(* Logix 5000 Controller export Example_PLC; controller Example_PLC 1769-L32E rev 19.11; software revision 19.01; part 6 of 6 *)

ADD_ON_INSTRUCTION AKD_Stop_Smooth   (* revision 2.3, ExecutePrescan, ExecuteEnableInFalse *)
// Motion Smooth Stop
// Revision note:
// Remove the command timeout (allow unlimited time to stop). Add an IP In Progress bit which is active while stopping.
VAR_OUTPUT
   DN : BOOL; {access Read Only, visible}   // Command Successful
   ER : BOOL; {access Read Only, visible}   // Error
END_VAR
VAR_IN_OUT
   Axis : AKD_Axis; {required}
END_VAR
VAR_OUTPUT
   IP : BOOL; {access Read Only, visible}   // In Progress
END_VAR

ROUTINE EnableInFalse   (* ladder *)
// Enable In False
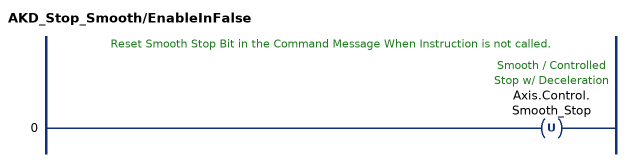
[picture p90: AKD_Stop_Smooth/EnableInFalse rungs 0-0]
   // Reset Smooth Stop Bit in the Command Message When Instruction is not called.
   0: OTU(Axis.Control.Smooth_Stop);
END_ROUTINE

ROUTINE Logic   (* ladder *)
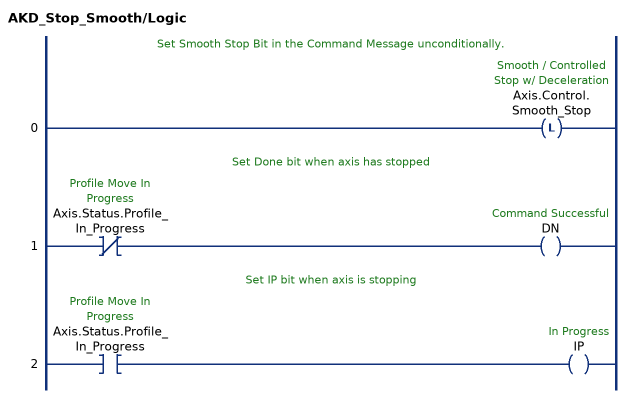
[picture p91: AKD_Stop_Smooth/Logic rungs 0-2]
   // Set Smooth Stop Bit in the Command Message unconditionally.
   0: OTL(Axis.Control.Smooth_Stop);
   // Set Done bit when axis has stopped
   1: XIO(Axis.Status.Profile_In_Progress)OTE(DN);
   // Set IP bit when axis is stopping
   2: XIC(Axis.Status.Profile_In_Progress)OTE(IP);
END_ROUTINE

ROUTINE Prescan   (* ladder *)
END_ROUTINE
END_ADD_ON_INSTRUCTION

ADD_ON_INSTRUCTION AKD_Torque_Move   (* revision 2.1, ExecutePrescan, ExecuteEnableInFalse *)
// Set Torque Command
VAR_OUTPUT
   DN : BOOL; {access Read Only, visible}   // Command Successful
   ER : BOOL; {access Read Only, visible}   // Error
END_VAR
VAR_IN_OUT
   Axis : AKD_Axis; {required}
END_VAR
VAR_INPUT
   Torque : DINT; {required}   // Torque Command
END_VAR
VAR
   Response_Bytes : SINT[8];
   OS_LoadStart : BOOL;
   Command_Timeout : TIMER := (PRE := 100);   // Timeout Timer
   Command_Message_Type : SINT;   // Command Message Type
   Command_Axis_Number : SINT;   // Command Axis Number
   Response_Message_Type : SINT;   // Response Message Type
   Response_Axis_Number : SINT;   // Response Axis Number
   Command_Bytes : SINT[8];
   Step : SINT;
END_VAR

ROUTINE EnableInFalse   (* ladder *)
// EnableIn_False
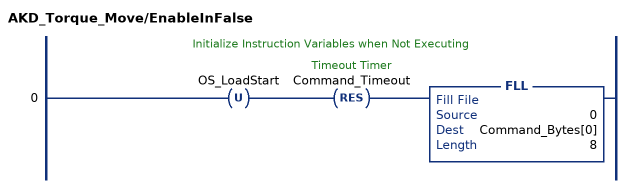
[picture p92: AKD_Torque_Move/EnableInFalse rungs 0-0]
   // Initialize Instruction Variables when Not Executing
   0: OTU(OS_LoadStart)RES(Command_Timeout)FLL(0,Command_Bytes[0],8);
END_ROUTINE

ROUTINE Logic   (* ladder *)
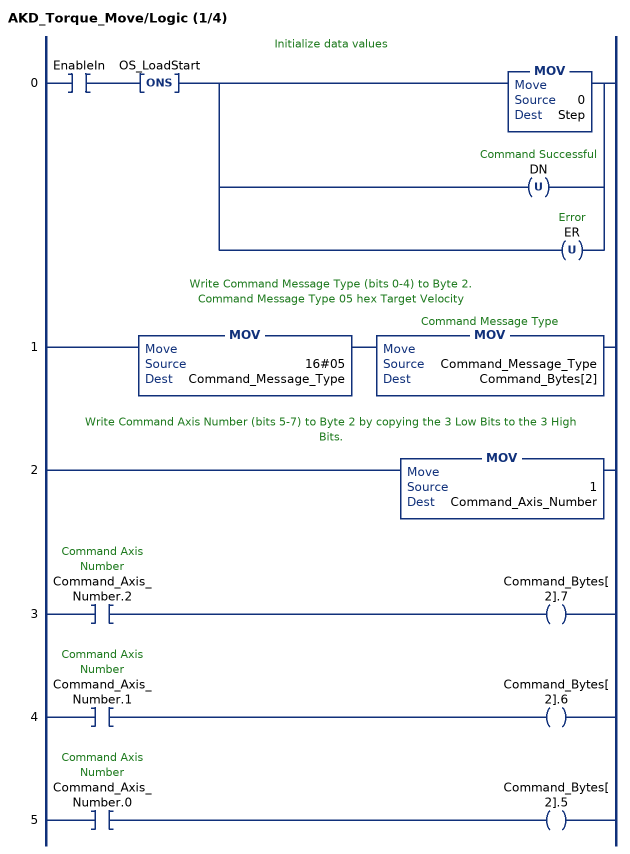
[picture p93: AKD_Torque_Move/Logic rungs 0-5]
   // Initialize data values
   0: XIC(EnableIn)ONS(OS_LoadStart)[MOV(0,Step) ,OTU(DN) ,OTU(ER) ];
   // Write Command Message Type (bits 0-4) to Byte 2.
   // Command Message Type 05 hex Target Velocity
   1: MOV(16#05,Command_Message_Type)MOV(Command_Message_Type,Command_Bytes[2]);
   // Write Command Axis Number (bits 5-7) to Byte 2 by copying the 3 Low Bits to the 3 High Bits.
   2: MOV(1,Command_Axis_Number);
   3: XIC(Command_Axis_Number.2)OTE(Command_Bytes[2].7);
   4: XIC(Command_Axis_Number.1)OTE(Command_Bytes[2].6);
   5: XIC(Command_Axis_Number.0)OTE(Command_Bytes[2].5);
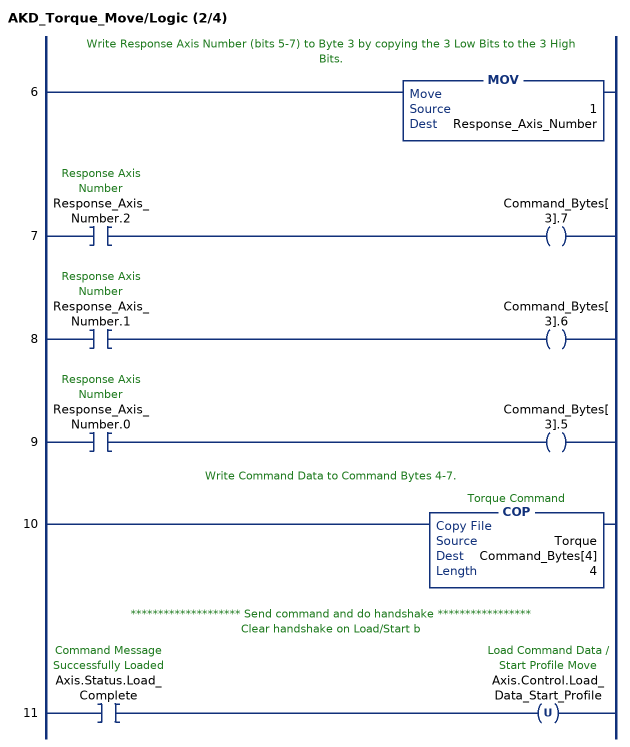
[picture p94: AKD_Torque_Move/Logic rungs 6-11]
   // Write Response Axis Number (bits 5-7) to Byte 3 by copying the 3 Low Bits to the 3 High Bits.
   6: MOV(1,Response_Axis_Number);
   7: XIC(Response_Axis_Number.2)OTE(Command_Bytes[3].7);
   8: XIC(Response_Axis_Number.1)OTE(Command_Bytes[3].6);
   9: XIC(Response_Axis_Number.0)OTE(Command_Bytes[3].5);
   // Write Command Data to Command Bytes 4-7.
   10: COP(Torque,Command_Bytes[4],4);
   // ******************** Send command and do handshake *****************
   // Clear handshake on Load/Start b
   11: XIC(Axis.Status.Load_Complete)OTU(Axis.Control.Load_Data_Start_Profile);
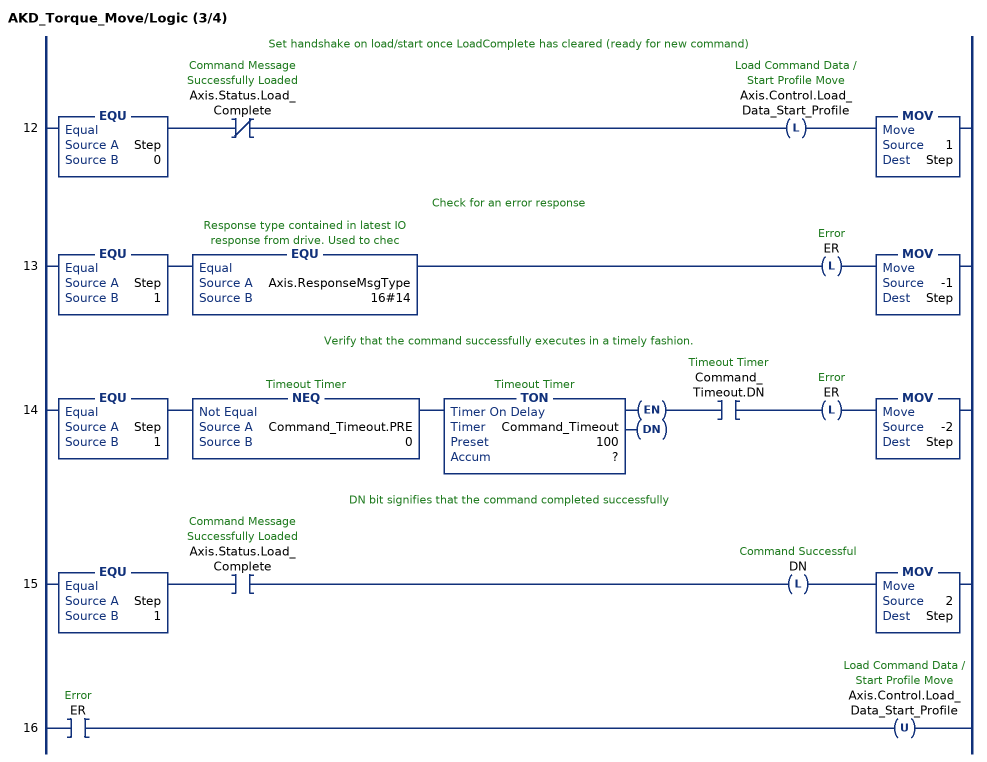
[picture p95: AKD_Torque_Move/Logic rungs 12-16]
   // Set handshake on load/start once LoadComplete has cleared (ready for new command)
   12: EQU(Step,0)XIO(Axis.Status.Load_Complete)OTL(Axis.Control.Load_Data_Start_Profile)MOV(1,Step);
   // Check for an error response
   13: EQU(Step,1)EQU(Axis.ResponseMsgType,16#14)OTL(ER)MOV(-1,Step);
   // Verify that the command successfully executes in a timely fashion.
   14: EQU(Step,1)NEQ(Command_Timeout.PRE,0)TON(Command_Timeout,?,?)XIC(Command_Timeout.DN)OTL(ER)MOV(-2,Step);
   // DN bit signifies that the command completed successfully
   15: EQU(Step,1)XIC(Axis.Status.Load_Complete)OTL(DN)MOV(2,Step);
   16: XIC(ER)OTU(Axis.Control.Load_Data_Start_Profile);
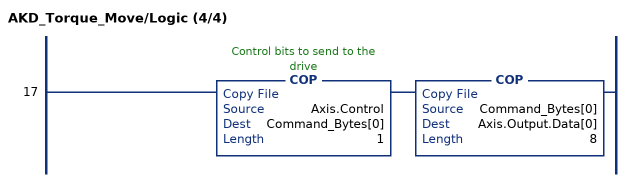
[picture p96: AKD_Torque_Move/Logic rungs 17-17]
   17: COP(Axis.Control,Command_Bytes[0],1)COP(Command_Bytes[0],Axis.Output.Data[0],8);
END_ROUTINE

ROUTINE Prescan   (* ladder *)
// Prescan
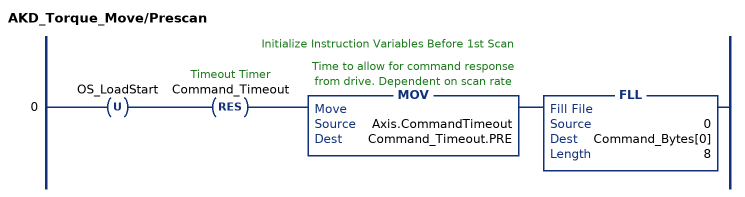
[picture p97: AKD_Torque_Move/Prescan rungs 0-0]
   // Initialize Instruction Variables Before 1st Scan
   0: OTU(OS_LoadStart)RES(Command_Timeout)MOV(Axis.CommandTimeout,Command_Timeout.PRE)FLL(0,Command_Bytes[0],8);
END_ROUTINE
END_ADD_ON_INSTRUCTION

VAR_GLOBAL   (* controller tags *)
   AIN_VALUE : DINT := 7047;
   AKD_1 : AKD_Drive;
   AOUT : DINT;
   AOUT_VALUEU : LINT;
   Axis_1 : AKD_Drive;
   AXIS_ONE : AKD_Axis := (Status.Current_Direction := 1, Input.Data[0] := 16, Input.Data[8] := -6, Input.Data[9] := 78, Input.Data[12] := -19, Input.Data[13] := 10, PositionFeedback := 20218, VelocityFeedback := 2797);
   DIN1_STATE : BOOL;
   DM_EN_SET : BOOL := 1;
   DOUT_STATEU : BOOL;
   Dynamic : BOOL;
   EN : BOOL;
   OneShot : BOOL;
   Start_Dynamic_data_transfer : BOOL;
   Start_Dynamic_mapped_Data : BOOL;
END_VAR

PROGRAM MainProgram   (* main routine MainRoutine *)

ROUTINE MainRoutine   (* ladder *)
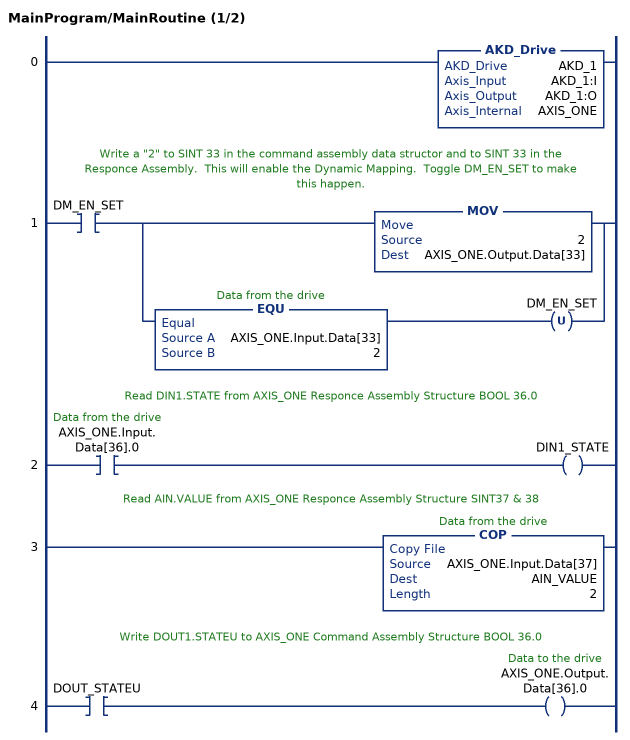
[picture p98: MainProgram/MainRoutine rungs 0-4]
   0: AKD_Drive(AKD_1,AKD_1:I,AKD_1:O,AXIS_ONE);
   // Write a "2" to SINT 33 in the command assembly data structor and to SINT 33 in the Responce Assembly.  This will enable the Dynamic Mapping.  Toggle DM_EN_SET to make this happen.
   1: XIC(DM_EN_SET)[MOV(2,AXIS_ONE.Output.Data[33]) ,EQU(AXIS_ONE.Input.Data[33],2) OTU(DM_EN_SET) ];
   // Read DIN1.STATE from AXIS_ONE Responce Assembly Structure BOOL 36.0
   2: XIC(AXIS_ONE.Input.Data[36].0)OTE(DIN1_STATE);
   // Read AIN.VALUE from AXIS_ONE Responce Assembly Structure SINT37 & 38
   3: COP(AXIS_ONE.Input.Data[37],AIN_VALUE,2);
   // Write DOUT1.STATEU to AXIS_ONE Command Assembly Structure BOOL 36.0
   4: XIC(DOUT_STATEU)OTE(AXIS_ONE.Output.Data[36].0);
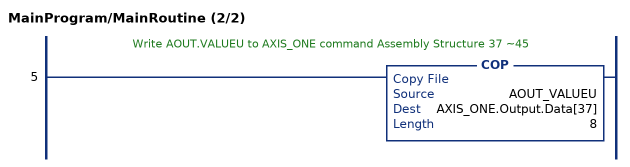
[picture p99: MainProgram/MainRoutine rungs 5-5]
   // Write AOUT.VALUEU to AXIS_ONE command Assembly Structure 37 ~45
   5: COP(AOUT_VALUEU,AXIS_ONE.Output.Data[37],8);
END_ROUTINE
END_PROGRAM
